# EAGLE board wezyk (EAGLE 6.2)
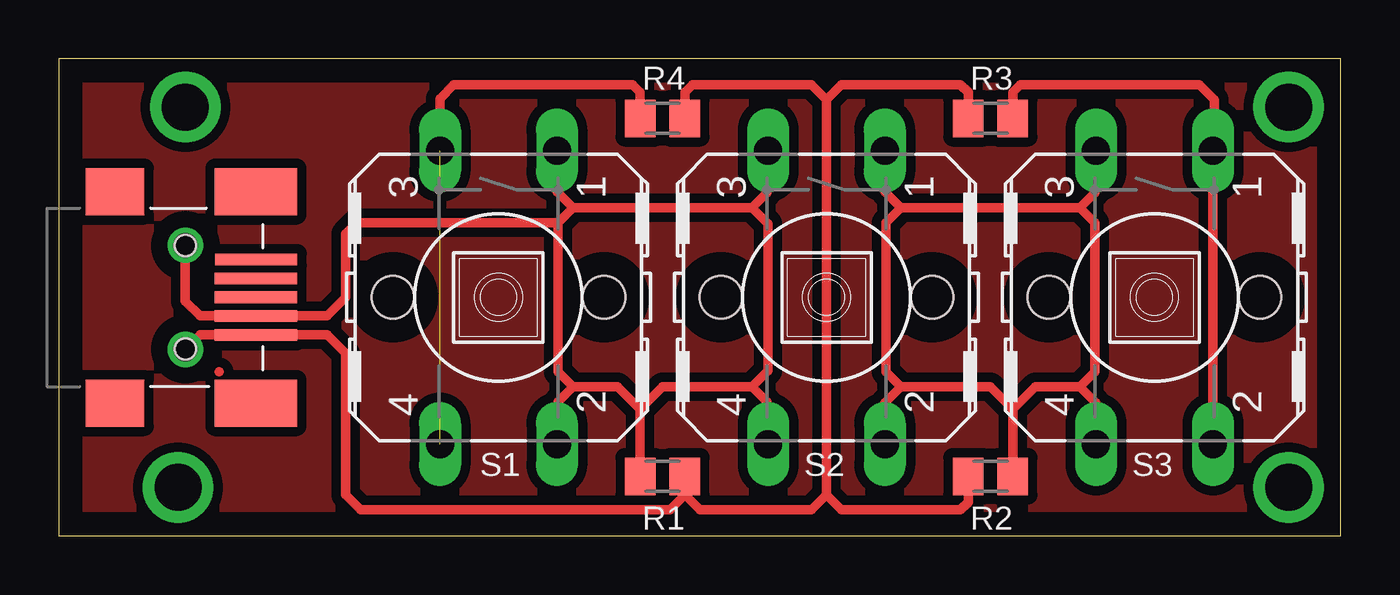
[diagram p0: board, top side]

Size 54.61 x 20.32 mm. Coordinates in mm from the lower left corner, seen from the top.
Outline: 0,0 54.61,0 54.61,20.32 0,20.32 0,0
Copper layers (1*16): Top 0.035mm / dielectric 1.5mm / Bottom 0.035mm
Design rules: minimum track width 10mil, minimum drill 24mil, track to track 8mil, track to pad 8mil, pad to pad 8mil, via to via 8mil, smd to smd 8mil, copper to edge 40mil, drill to drill 8mil, minimum pad ring 10mil, minimum via ring 8mil, stop-mask expansion 4mil, vias tented up to drill 0mil, thermal gap 10mil

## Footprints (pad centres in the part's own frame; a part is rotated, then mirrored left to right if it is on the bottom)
M0805 = smd 1.3 x 1.6: 1 -0.95,0; 2 0.95,0
B3F-40XX = drill 1.194 long: 1 -6.248,2.489; 2 6.248,2.489; 3 -6.248,-2.489; 4 6.248,-2.489 | hole 1.803: 0,-4.496; 0,4.496
USB-MINIB-OLD = smd 2.5 x 2: 1 -3,-4.5; 2 -3,4.5 | smd 3.5 x 2: 3 3,-4.5; 4 3,4.5 | smd 3.5 x 0.5: D+ 3,0; D- 3,0.8; GND 3,-1.6; ID 3,-0.8; VBUS 3.01,1.61 | hole 0.9: 0,2.2; 0,-2.2

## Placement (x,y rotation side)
R1  82k  [M0805]  25.72,2.54 180 top
R2  39k  [M0805]  39.69,2.54 0 top
R3  12k  [M0805]  39.69,17.78 0 top
R4  8,2k  [M0805]  25.72,17.78 180 top
S1  [B3F-40XX]  18.73,10.16 270 top
S2  [B3F-40XX]  32.7,10.16 270 top
S3  [B3F-40XX]  46.67,10.16 270 top
X1  USBOLD  [USB-MINIB-OLD]  5.4,10.16 0 top

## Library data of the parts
R1-R4 = rcl
S1-S3 = switch-omron; MF: OMRON COMPONENTS USA; MPN: B3F-4000; OC_FARNELL: 176434; OC_NEWARK: 36K3105
X1 = SparkFun

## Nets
N$1: R1.2 S1.1 S1.2 S2.3 S2.4
N$2: R2.2 S2.1 S2.2 S3.3 S3.4
N$3: R3.2 S3.1 S3.2
N$4: R1.1 R2.1 R3.1 R4.1 X1.GND
N$5: R4.2 S1.3 S1.4

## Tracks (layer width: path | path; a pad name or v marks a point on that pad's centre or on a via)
123
  pour Top (isolate 0.406): -0.32,20.8 -0.32,-0.48 54.93,-0.48 54.93,20.8
N$1
  Top 0.406: S2.4 30.21,5.03 30.16,5.08 30.16,5.71 29.53,6.35 | 24.77,5.39 R1.2 | 24.77,5.39 23.81,6.35 21.91,6.35 | 21.91,6.35 21.27,5.71 21.27,3.96 S1.2 | 24.77,5.39 24.77,5.4 25.72,6.35 29.53,6.35 | 29.53,6.35 30.21,7.04 30.21,13.28 29.53,13.97 | S1.1 21.22,14.66 21.91,13.97 | 21.91,13.97 29.53,13.97 | 29.53,13.97 30.16,14.6 30.16,16.36 S2.3 | 21.27,13.34 21.91,13.97 | 21.91,6.35 21.27,6.98 21.27,13.34 | 5.4,12.38 5.4,10 6.03,9.37 11.43,9.37 12.22,10.16 12.22,12.86 12.7,13.34 21.27,13.34
N$2
  Top 0.406: S2.2 35.19,5.66 35.88,6.35 | 35.88,6.35 39.69,6.35 40.64,5.4 | 40.64,5.4 R2.2 | S2.1 35.19,14.66 35.88,13.97 | 35.88,13.97 43.5,13.97 | 43.5,13.97 44.13,14.6 44.13,16.36 S3.3 | 35.88,6.35 35.24,6.98 35.24,13.34 35.88,13.97 | S3.4 44.18,5.66 43.5,6.35 | 43.5,6.35 41.59,6.35 40.64,5.4 | 43.5,13.97 44.13,13.34 44.13,6.98 43.5,6.35
N$3
  Top 0.406: S3.2 S3.1 49.21,16.46 49.21,18.57 48.58,19.21 40.96,19.21 40.64,18.89 R3.2
N$4
  Top 0.406: R4.1 26.67,18.89 26.99,19.21 32.07,19.21 32.7,18.57 | 26.67,1.75 27.31,1.11 32.07,1.11 32.7,1.75 | R2.1 38.74,1.43 38.42,1.11 33.34,1.11 32.7,1.75 | R3.1 38.74,18.89 38.42,19.21 33.34,19.21 32.7,18.57 | 32.7,1.75 32.7,18.57 | 26.67,1.75 26.67,1.74 26.03,1.11 12.86,1.11 12.22,1.75 12.22,7.78 11.44,8.56 X1.GND 6.02,8.56 5.4,7.94 | 26.67,1.75 R1.1
N$5  (1 unrouted)
  Top 0.406: R4.2 24.77,18.89 24.45,19.21 16.83,19.21 16.24,18.62 S1.3
N$6  (via drill 1)
  other vias: 5.4,12.38
N$7  (via drill 1)
  other vias: 5.4,7.94
N$8  (via drill 2)
  other vias: 5.4,18.26
N$9  (via drill 2)
  other vias: 5.08,2.06
N$10  (via drill 2)
  other vias: 52.39,18.26
N$11  (via drill 2)
  other vias: 52.39,2.06
N$12
  Top 0.406: 6.83,6.98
